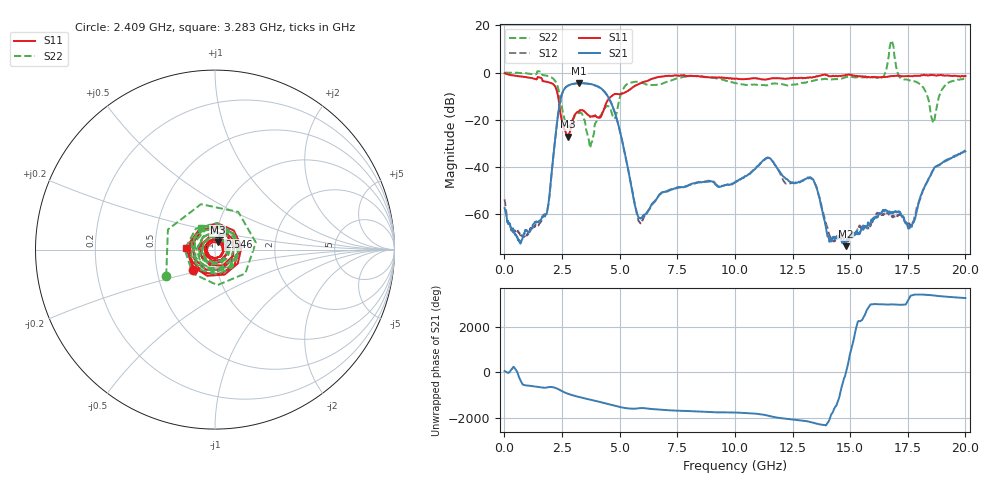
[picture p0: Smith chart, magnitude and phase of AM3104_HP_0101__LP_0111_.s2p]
!Created with skrf (http://scikit-rf.org).
# Hz S RI R 50.0
!freq ReS11 ImS11 ReS21 ImS21 ReS12 ImS12 ReS22 ImS22
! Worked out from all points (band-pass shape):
!   1601 points, 10 MHz to 20 GHz, reference 50 ohm
!   highest |S21| = -4.52 dB at 3.246 GHz (marker M1); lowest = -73.7 dB at 14.8 GHz (marker M2)
!   |S21| within 3 dB of the highest: 2.566 GHz to 4.288 GHz (1.722 GHz wide, 50.2 % of centre)
!   lowest |S11| = -27.3 dB at 2.759 GHz (marker M3), VSWR 1.09, Z = 51.4 + j4.16 ohm
!   |S11| at or under -10 dB: 2.327 GHz to 4.651 GHz (2.324 GHz wide, 66.6 % of centre)
!   |S22| runs from -32.0 to 13.6 dB; largest |S21 - S12| = 0.037
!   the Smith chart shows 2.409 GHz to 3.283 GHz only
!   S11 on the Smith chart (normalised r, x): 2.409 GHz: 0.77, -0.18; 2.546 GHz: 1.04, +0.15; 3.283 GHz: 0.72, +0.02
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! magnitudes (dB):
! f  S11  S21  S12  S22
! 10 MHz  -0.3  -57.5  -53.7  0.0
! 684.7 MHz  -1.7  -72.3  -69.0  -0.2
! 1.784 GHz  -3.8  -60.3  -60.2  -1.2
! 2.409 GHz  -15.7  -12.7  -12.7  -10.2
! 2.546 GHz  -22.5  -7.9  -7.9  -17.1
! 2.759 GHz  -27.3  -5.6  -5.6  -23.2
! 3.246 GHz  -16.5  -4.5  -4.6  -17.2
! 3.283 GHz  -15.9  -4.5  -4.6  -17.1
! 3.346 GHz  -16.0  -4.6  -4.6  -17.1
! 3.733 GHz  -18.8  -4.8  -4.9  -31.4
! 4.658 GHz  -10.0  -13.4  -13.6  -17.2
! 5.857 GHz  -4.8  -61.6  -63.3  -4.1
! 6.682 GHz  -1.9  -52.4  -52.5  -5.1
! 10.01 GHz  -2.7  -46.7  -46.7  -4.5
! 11.43 GHz  -2.8  -36.0  -36.2  -5.4
! 13.34 GHz  -2.1  -44.9  -45.1  -3.7
! 14.08 GHz  -1.5  -70.2  -68.1  -3.0
! 14.8 GHz  -1.1  -73.7  -71.5  -2.0
! 16.68 GHz  -1.6  -59.7  -60.3  7.2
! 17.6 GHz  -1.5  -65.1  -64.8  -3.4
! 18.6 GHz  -1.1  -41.5  -41.5  -21.3
! 20 GHz  -1.4  -33.5  -33.0  -2.5
